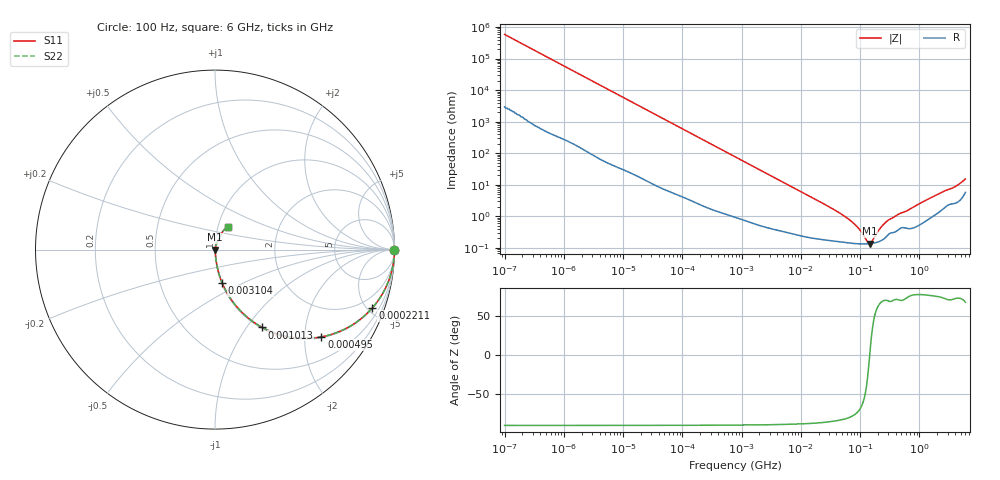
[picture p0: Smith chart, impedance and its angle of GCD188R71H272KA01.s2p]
!Murata Part Number: GCD188R71H272KA01
!These Parameters are Measured in Series Mode Connection
!Data Generated on Jan 08, 2026
!  o--ll--o
!Port1  Port2
!  o------o
!Operation Temp=25[degC], DC Bias Voltage=0[V]
!Freq. Start=100[Hz] Stop=6[GHz] 401[Steps]
# Hz S RI R 50
!Freq.(Hz) S11(Real) S11(Imag) S21(Real) S21(Imag) S12(Real) S12(Imag) S22(Real) S22(Imag)
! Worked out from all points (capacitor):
!   401 points, 100 Hz to 6 GHz, reference 50 ohm
!   read as one part in series: C = 2.73 nF near 109 Hz
!   lowest |Z| = 136 mohm at 145.9 MHz (marker M1)
!   series resonance near 145.4 MHz, so ESL is about 440 pH
!   S11 on the Smith chart (normalised r, x): 100 Hz: open; 221.1 kHz: 1.04, -5.39; 495 kHz: 1.02, -2.42; 1.013 MHz: 1.02, -1.19; 3.104 MHz: 1.01, -0.39; 6 GHz: 1.11, +0.28
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100  1 -0.000172  9e-07 0.000172  9e-07 0.000172  1 -0.000172
2008  1 -0.00342  2.81e-05 0.00342  2.81e-05 0.00342  1 -0.00342
40335  0.995 -0.0678  0.00501 0.0678  0.00501 0.0678  0.995 -0.0678
98762  0.972 -0.1615  0.028 0.1615  0.028 0.1615  0.972 -0.1615
221108  0.877 -0.3245  0.123 0.3245  0.123 0.3245  0.877 -0.3245
495019  0.5924 -0.4864  0.4076 0.4864  0.4076 0.4864  0.5924 -0.4864
774597  0.3761 -0.4784  0.6239 0.4784  0.6239 0.4784  0.3761 -0.4784
1013323  0.2628 -0.4336  0.7372 0.4336  0.7372 0.4336  0.2628 -0.4336
1658239  0.1205 -0.3178  0.8795 0.3178  0.8795 0.3178  0.1205 -0.3178
3103719  0.0403 -0.1864  0.9597 0.1864  0.9597 0.1864  0.0403 -0.1864
1.555665e7  0.00355 -0.039  0.9965 0.039  0.9965 0.039  0.00355 -0.039
3.983537e7  0.0018 -0.0145  0.9982 0.0145  0.9982 0.0145  0.0018 -0.0145
6.817316e7  0.00146 -0.00727  0.9985 0.00727  0.9985 0.00727  0.00146 -0.00727
9.326766e7  0.00136 -0.00404  0.9986 0.00404  0.9986 0.00404  0.00136 -0.00404
1.334425e8  0.00134 -0.000763  0.9987 0.000763  0.9987 0.000763  0.00134 -0.000763
1.459435e8  0.00136 3.56e-05  0.9986 -3.56e-05  0.9986 -3.56e-05  0.00136 3.56e-05
1.596157e8  0.00139 0.00084  0.9986 -0.00084  0.9986 -0.00084  0.00139 0.00084
2.283698e8  0.00171 0.00426  0.9983 -0.00426  0.9983 -0.00426  0.00171 0.00426
3.124326e8  0.00285 0.00736  0.9971 -0.00736  0.9971 -0.00736  0.00285 0.00736
1.497423e9  0.00965 0.0355  0.9904 -0.0355  0.9904 -0.0355  0.00965 0.0355
3.8344e9  0.0302 0.0746  0.9698 -0.0746  0.9698 -0.0746  0.0302 0.0746
6e9  0.0706 0.1245  0.9294 -0.1245  0.9294 -0.1245  0.0706 0.1245
